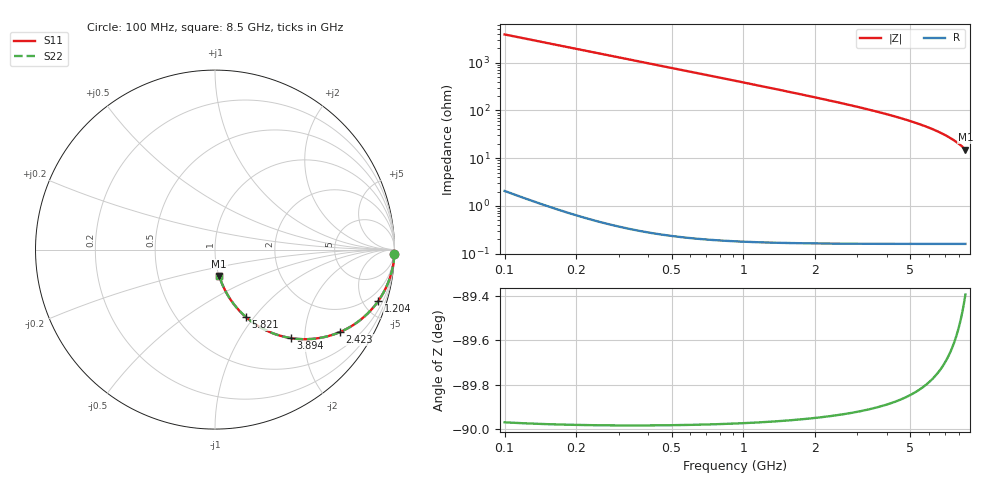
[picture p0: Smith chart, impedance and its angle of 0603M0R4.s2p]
! Created Wed Apr 18 11:53:04 2012
# hz S ma R 50
! 2 Port Network Data from SP1.SP block
! freq  magS11  angS11  magS21  angS21  magS12  angS12  magS22  angS22
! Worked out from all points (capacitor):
!   8401 points, 100 MHz to 8.5 GHz, reference 50 ohm
!   read as one part in series: C = 410 fF near 142 MHz
!   lowest |Z| = 15.1 ohm at 8.5 GHz (marker M1)
!   S11 on the Smith chart (normalised r, x): 100 MHz: 1, -78; 1.204 GHz: 1.00, -6.36; 2.423 GHz: 1.00, -3.03; 3.894 GHz: 1.00, -1.71; 5.821 GHz: 1.00, -0.92; 8.5 GHz: 1.00, -0.30
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1e8  0.9997 -1.5  0.02575 88.5  0.02575 88.5  0.9997 -1.5
1.24e8  0.9995 -1.8  0.03193 88.1  0.03193 88.1  0.9995 -1.8
1.88e8  0.9988 -2.8  0.04839 87.2  0.04839 87.2  0.9988 -2.8
2.55e8  0.9978 -3.8  0.06559 86.2  0.06559 86.2  0.9978 -3.8
3.49e8  0.9959 -5.1  0.08964 84.8  0.08964 84.8  0.9959 -5.1
4.64e8  0.9929 -6.8  0.1189 83.2  0.1189 83.2  0.9929 -6.8
6.07e8  0.9879 -8.9  0.155 81.1  0.155 81.1  0.9879 -8.9
7.77e8  0.9803 -11.4  0.1973 78.6  0.1973 78.6  0.9803 -11.4
9.75e8  0.9693 -14.2  0.2456 75.8  0.2456 75.8  0.9693 -14.2
1.204e9  0.9538 -17.4  0.2999 72.5  0.2999 72.5  0.9538 -17.4
1.5e9  0.93 -21.5  0.367 68.4  0.367 68.4  0.93 -21.5
1.927e9  0.8891 -27.2  0.457 62.8  0.457 62.8  0.8891 -27.2
2.423e9  0.8342 -33.4  0.5506 56.5  0.5506 56.5  0.8342 -33.4
2.9e9  0.7765 -39.0  0.6291 50.9  0.6291 50.9  0.7765 -39.0
3.894e9  0.6501 -49.3  0.7586 40.6  0.7586 40.6  0.6501 -49.3
4.3e9  0.5985 -53.1  0.7998 36.8  0.7998 36.8  0.5985 -53.1
4.993e9  0.5127 -59.0  0.8572 30.8  0.8572 30.8  0.5127 -59.0
5.7e9  0.4294 -64.4  0.9017 25.4  0.9017 25.4  0.4294 -64.4
5.821e9  0.4157 -65.2  0.9081 24.6  0.9081 24.6  0.4157 -65.2
7.1e9  0.2795 -73.5  0.9586 16.2  0.9586 16.2  0.2795 -73.5
7.836e9  0.2087 -77.5  0.9764 12.0  0.9764 12.0  0.2087 -77.5
8.5e9  0.1491 -80.8  0.9872 8.6  0.9872 8.6  0.1491 -80.8
